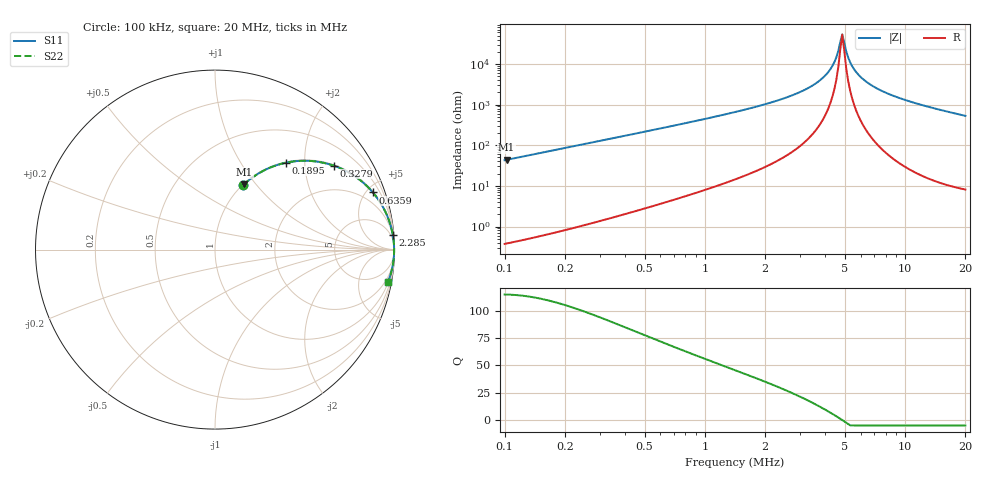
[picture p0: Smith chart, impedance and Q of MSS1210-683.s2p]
# MHz S MA R 50
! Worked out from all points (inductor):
!   233 points, 100 kHz to 20 MHz, reference 50 ohm
!   read as one part in series: L = 68 uH near 102.3 kHz
!   highest Q = 115 at 102.3 kHz (marker M1), where L = 68 uH
!   self-resonance near 4.744 MHz
!   S11 on the Smith chart (normalised r, x): 100 kHz: 1.01, +0.85; 189.5 kHz: 1.02, +1.62; 327.9 kHz: 1.03, +2.81; 635.9 kHz: 1.08, +5.50; 2.285 MHz: 2, +25; 20 MHz: 1, -11
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0.1  0.3918 66.4  0.9166 -23.1  0.9166 -23.1  0.3918 66.4
0.10231  0.3994 66.0  0.9133 -23.5  0.9133 -23.5  0.3994 66.0
0.1895442  0.6264 50.7  0.7737 -38.8  0.7737 -38.8  0.6264 50.7
0.2436751  0.7176 43.6  0.6893 -45.9  0.6893 -45.9  0.7176 43.6
0.327905  0.8101 35.3  0.5775 -54.1  0.5775 -54.1  0.8101 35.3
0.5937753  0.9272 21.2  0.3618 -68.0  0.3618 -68.0  0.9272 21.2
0.6358825  0.9355 19.9  0.3402 -69.3  0.3402 -69.3  0.9355 19.9
1.446882  0.986 8.4  0.1464 -80.3  0.1464 -80.3  0.986 8.4
2.284535  0.9942 4.6  0.07996 -83.6  0.07996 -83.6  0.9942 4.6
3.446086  0.9973 1.9  0.03393 -84.4  0.03393 -84.4  0.9973 1.9
3.952169  0.9978 1.1  0.02016 -83.1  0.02016 -83.1  0.9978 1.1
4.330204  0.998 0.6  0.01124 -79.3  0.01124 -79.3  0.998 0.6
4.532574  0.9981 0.4  0.006887 -73.4  0.006887 -73.4  0.9981 0.4
4.853998  0.9981 -0.0  0.001876 1.6  0.001876 1.6  0.9981 -0.0
5.080846  0.9981 -0.3  0.004858 67.4  0.004858 67.4  0.9981 -0.3
5.198215  0.9981 -0.4  0.006964 74.4  0.006964 74.4  0.9981 -0.4
5.44115  0.9981 -0.6  0.01132 80.2  0.01132 80.2  0.9981 -0.6
5.695439  0.9981 -0.9  0.01576 82.6  0.01576 82.6  0.9981 -0.9
6.682744  0.9978 -1.8  0.03172 85.1  0.03172 85.1  0.9978 -1.8
8.397251  0.9967 -3.2  0.05604 85.1  0.05604 85.1  0.9967 -3.2
12.10121  0.993 -5.8  0.1013 83.1  0.1013 83.1  0.993 -5.8
20  0.9798 -10.7  0.1854 78.4  0.1854 78.4  0.9798 -10.7
